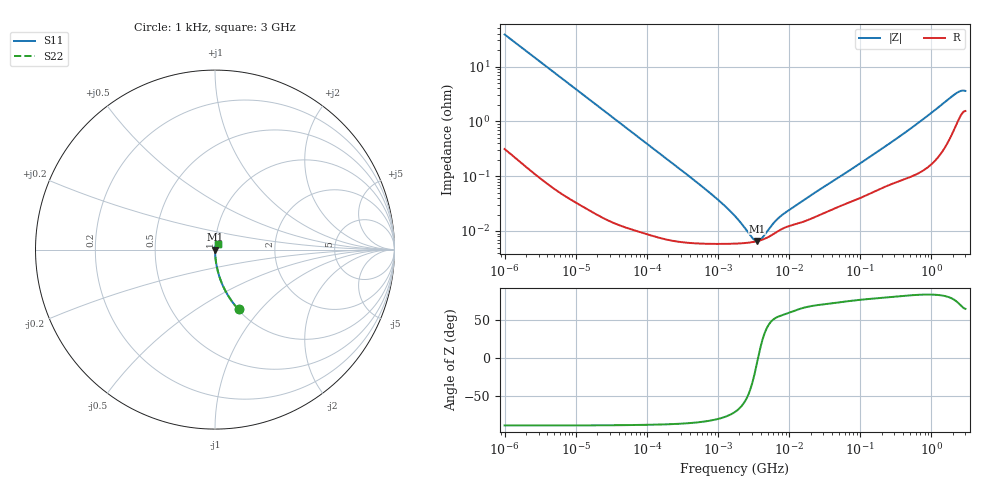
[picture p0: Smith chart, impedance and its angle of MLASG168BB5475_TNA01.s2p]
! MLASG168BB5475_TNA01  S-PARAMETER MODEL  ( Standard Model )
! Model Generated by TAIYO YUDEN Corporation (http://www.ty-top.com)
! Version 1.0
! TAIYO YUDEN Control No. 220601
! Copyright(c) 2019 TAIYO YUDEN CO.,LTD. All Rights Reserved.
! Product Description (link to TY-COMPAS)
! https://ds.yuden.co.jp/TYCOMPAS/or/detail?pn=MLASG168BB5475KTNA01&u=M
! Products Name : Multilayer Ceramic Capacitors
! Characteristics :
!  Capacitance : 4.7 [uF] , Rated Voltage : 35 [V] , TCC : X5R
!  Case Size : 1.6 x 0.8 / 0.063 x 0.031 [mm/inch] , Thickness : 0.8 / 0.031 [mm/inch]
!  (Conditions: Temperature = 25 [degC] , DC Bias Voltage = 0 [V])
! External Node Assignments :
!  1  o---| |---o  2
! GND o---------o GND
! Frequency Range : 1kHz  -  3GHz  [ 401 STEP ]
# MHZ S RI R 50
! Freq[MHz].  S11 Real  S11 Imag  S21 Real  S21 Imag  S12 Real  S12 Imag  S22 Real  S22 Imag
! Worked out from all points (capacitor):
!   401 points, 1 kHz to 3 GHz, reference 50 ohm
!   read as one part in series: C = 4.13 uF near 1.077 kHz
!   lowest |Z| = 6.57 mohm at 3.517 MHz (marker M1)
!   series resonance near 3.662 MHz, so ESL is about 460 pH
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0.001  0.131 -0.3334  0.869 0.3334  0.869 0.3334  0.131 -0.3334
0.001685  0.0514 -0.2169  0.9486 0.2169  0.9486 0.2169  0.0514 -0.2169
0.00306  0.0166 -0.1242  0.9834 0.1242  0.9834 0.1242  0.0166 -0.1242
0.005768  0.00501 -0.0669  0.995 0.0669  0.995 0.0669  0.00501 -0.0669
0.01216  0.00131 -0.032  0.9987 0.032  0.9987 0.032  0.00131 -0.032
0.147855  8.26e-05 -0.00266  0.9999 0.00266  0.9999 0.00266  8.26e-05 -0.00266
0.791611  5.85e-05 -0.000477  0.9999 0.000477  0.9999 0.000477  5.85e-05 -0.000477
1.238299  5.83e-05 -0.000284  0.9999 0.000284  0.9999 0.000284  5.83e-05 -0.000284
1.732051  5.89e-05 -0.000178  0.9999 0.000178  0.9999 0.000178  5.89e-05 -0.000178
2.514714  6.08e-05 -8.36e-05  0.9999 8.36e-05  0.9999 8.36e-05  6.08e-05 -8.36e-05
2.812335  6.18e-05 -5.81e-05  0.9999 5.81e-05  0.9999 5.81e-05  6.18e-05 -5.81e-05
3.517417  6.51e-05 -8.76e-06  0.9999 8.76e-06  0.9999 8.76e-06  6.51e-05 -8.76e-06
4.566395  7.26e-05 4.8e-05  0.9999 -4.8e-05  0.9999 -4.8e-05  7.26e-05 4.8e-05
4.919932  7.59e-05 6.42e-05  0.9999 -6.42e-05  0.9999 -6.42e-05  7.59e-05 6.42e-05
6.629817  9.54e-05 0.000127  0.9999 -0.000127  0.9999 -0.000127  9.54e-05 0.000127
7.988506  0.00011 0.000164  0.9999 -0.000164  0.9999 -0.000164  0.00011 0.000164
21.06097  0.000171 0.000432  0.9998 -0.000432  0.9998 -0.000432  0.000171 0.000432
256.0921  0.000707 0.00387  0.9993 -0.00387  0.9993 -0.00387  0.000707 0.00387
650.4536  0.00121 0.00927  0.9988 -0.00927  0.9988 -0.00927  0.00121 0.00927
2144.796  0.00856 0.03  0.9914 -0.03  0.9914 -0.03  0.00856 0.03
2584.342  0.0138 0.0327  0.9862 -0.0327  0.9862 -0.0327  0.0138 0.0327
3000  0.0162 0.0315  0.9838 -0.0315  0.9838 -0.0315  0.0162 0.0315
